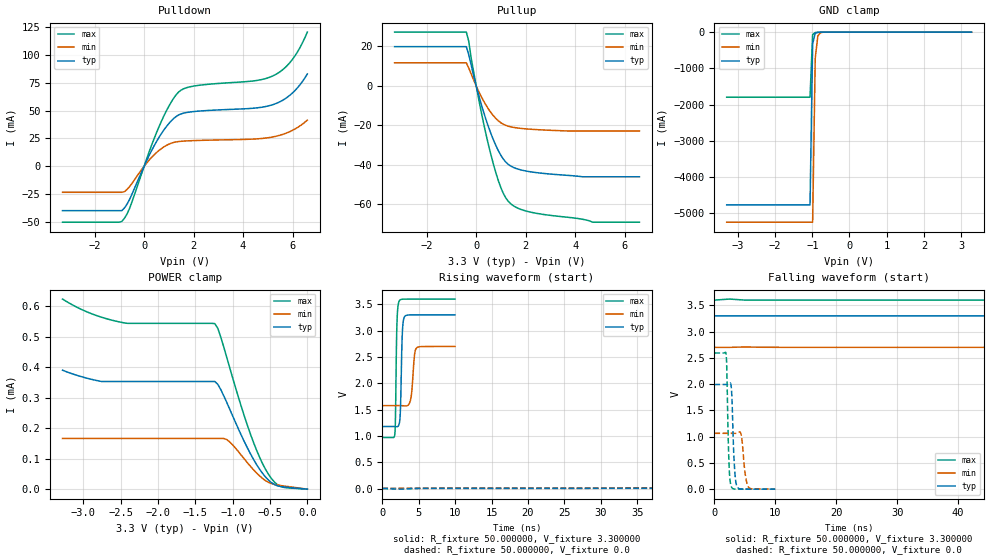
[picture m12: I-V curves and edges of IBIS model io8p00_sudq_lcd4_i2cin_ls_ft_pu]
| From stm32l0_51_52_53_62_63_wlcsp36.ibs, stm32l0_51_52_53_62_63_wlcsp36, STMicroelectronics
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|   Model io8p00_sudq_lcd4_i2cin_ls_ft_pu
[Model]  io8p00_sudq_lcd4_i2cin_ls_ft_pu
Model_type I/O
Polarity   Non-Inverting
Enable   Active-Low
Vinl =   0.990000V
Vinh =   2.310000V
Vmeas =  1.650000V
Cref =   50.000000pF
Rref =   100.000000M
Vref =   0.0V
C_comp   2.499500pF   2.460800pF   2.557800pF
[Temperature Range]   25.000000   0.125000k   -40.000000
[Pullup Reference]   3.300000V   2.700000V   3.600000V
[Pulldown Reference]   0.0V   0.0V   0.0V
[POWER Clamp Reference]   3.300000V   2.700000V   3.600000V
[GND Clamp Reference]   0.0V   0.0V   0.0V
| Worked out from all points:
|   slope of the pulldown table from 0 to 0.495 V, typ, clamps not added: 22.6 ohm
|   slope of the pullup table from 0 to 0.495 V, typ, clamps not added: 23.9 ohm
|   GND clamp passes 1 mA (typ) near -0.64 V on its own axis
|   rising waveform, R_fixture 50.000000, V_fixture 3.300000: 20-80 % time 216ps typ, 364ps min, 175ps max; typ from 1.18 V to 3.3 V
|   rising waveform, R_fixture 50.000000, V_fixture 0.0: 20-80 % time 204ns typ, 424ns min, 99.3ns max; typ from 0.001 V to 1.99 V
|   falling waveform, R_fixture 50.000000, V_fixture 3.300000: 20-80 % time 192ns typ, 381ns min, 105ns max; typ from 3.3 V to 1.18 V
|   falling waveform, R_fixture 50.000000, V_fixture 0.0: 20-80 % time 387ps typ, 554ps min, 311ps max; typ from 1.99 V to 0.001 V
[Pulldown]
|Voltage   I(typ)   I(min)   I(max)
-3.3V     -39.83mA   -23.36mA   -50.2mA
-900mV    -39.83mA   -23.36mA   -49.52mA
-600mV    -30.28mA   -18.59mA   -38.45mA
100mV     4.867mA    2.821mA    6.48mA
600mV     25.85mA    14.17mA    35.39mA
1V        38.33mA    19.81mA    53.88mA
1.4V      46.1mA     22.18mA    66.72mA
2V        49.07mA    23.02mA    71.93mA
4.5V      52.25mA    24.5mA     76.81mA
5.2V      55.25mA    26.31mA    81.02mA
6V        65.79mA    32.24mA    95.96mA
6.6V      82.83mA    41.41mA    120.4mA
[Pullup]
|Voltage   I(typ)   I(min)   I(max)
-3.3V     19.9mA     11.73mA    27.27mA
-400mV    19.9mA     11.73mA    27.27mA
-300mV    15.74mA    8.978mA    22.52mA
-200mV    10.44mA    5.968mA    13.84mA
200mV     -9.115mA   -5.294mA   -12.98mA
600mV     -24.29mA   -13.56mA   -35.12mA
1V        -35.2mA    -18.69mA   -51.63mA
1.2V      -38.62mA   -19.99mA   -56.79mA
1.4V      -40.6mA    -20.72mA   -59.71mA
2.2V      -43.48mA   -21.92mA   -63.91mA
4.7V      -46mA      -22.8mA    -69mA
6.6V      -46mA      -22.8mA    -69mA
[GND_clamp]
|Voltage   I(typ)   I(min)   I(max)
-3.3V     -4.766A    -5.244A    -1.797A
-1.06V    -4.766A    -5.244A    -1.797A
-990mV    -326.4mA   -5.244A    -67.85mA
-920mV    -28.83mA   -721.7mA   -11.08mA
-850mV    -6.686mA   -104.1mA   -6.707mA
-780mV    -3.552mA   -17.28mA   -4.326mA
-500mV    -59.41uA   -172uA     -34.91uA
3.28V     0A         0A         0A
[POWER_clamp]
|Voltage   I(typ)   I(min)   I(max)
-3.28V    390.5uA    166.4uA    624.1uA
-2.76V    353.6uA    166.4uA    564.7uA
-2.44V    353.6uA    166.4uA    545.3uA
-1.24V    353.6uA    166.4uA    543.5uA
-1.2V     344.2uA    166.4uA    528.2uA
-1.16V    327.1uA    166.4uA    499.5uA
-1.04V    262.6uA    155.2uA    398.8uA
-760mV    115.1uA    74.4uA     179.3uA
-560mV    39.87uA    27.94uA    65.07uA
-440mV    15uA       15.53uA    23.15uA
-360mV    8.745uA    12.05uA    9.091uA
0V        0A         0A         0A
[Ramp]
| variable   typ   min   max
dV/dt_r  1.19492/0.20344u   0.61283/0.42621u   1.55547/99.16188n
dV/dt_f  1.27224/0.19134u   0.63582/0.38119u   1.57816/0.10502u
R_load = 50.000000
[Rising Waveform]
R_fixture= 50.000000
V_fixture= 3.300000
V_fixture_min= 2.700000
V_fixture_max= 3.600000
|time   V(typ)   V(min)   V(max)
0s        1.178V     1.575V     969.7mV
1.702ns   1.177V     1.575V     1.018V
2.002ns   1.174V     1.575V     3.123V
2.322ns   1.235V     1.575V     3.563V
2.482ns   1.505V     1.576V     3.587V
2.743ns   2.948V     1.574V     3.597V
3.003ns   3.253V     1.571V     3.598V
3.884ns   3.299V     1.691V     3.599V
4.725ns   3.3V       2.675V     3.6V
9.97ns    3.3V       2.7V       3.6V
[Rising Waveform]
R_fixture= 50.000000
V_fixture= 0.0
V_fixture_min= 0.0
V_fixture_max= 0.0
|time   V(typ)   V(min)   V(max)
0s        1.061mV    1.817mV    656.1uV
50.05ns   4.344mV    4.548mV    94.15mV
100.1ns   82.31mV    4.577mV    928.9mV
165.2ns   466.8mV    10.16mV    1.944V
205.2ns   757.5mV    21.01mV    2.299V
252.8ns   1.082V     58.36mV    2.483V
362.9ns   1.608V     205.7mV    2.576V
503ns     1.883V     450.2mV    2.591V
878.4ns   1.99V      923.1mV    2.593V
1.246us   1.993V     1.064V     2.593V
[Falling Waveform]
R_fixture= 50.000000
V_fixture= 3.300000
V_fixture_min= 2.700000
V_fixture_max= 3.600000
|time   V(typ)   V(min)   V(max)
0s        3.3V       2.7V       3.6V
82.58ns   3.3V       2.7V       3.49V
150.2ns   3.19V      2.7V       2.488V
212.7ns   2.837V     2.697V     1.577V
247.7ns   2.596V     2.687V     1.236V
285.3ns   2.326V     2.665V     1.083V
390.4ns   1.64V      2.552V     998.5mV
490.5ns   1.343V     2.387V     980mV
868.4ns   1.192V     1.749V     970.2mV
1.246us   1.178V     1.575V     969.7mV
[Falling Waveform]
R_fixture= 50.000000
V_fixture= 0.0
V_fixture_min= 0.0
V_fixture_max= 0.0
|time   V(typ)   V(min)   V(max)
0s        1.993V     1.064V     2.593V
1.922ns   1.993V     1.064V     2.563V
2.022ns   1.992V     1.064V     2.306V
2.382ns   1.997V     1.064V     508.3mV
2.783ns   1.914V     1.064V     46.19mV
3.243ns   511.2mV    1.064V     4.312mV
3.664ns   62.27mV    1.066V     1.499mV
4.384ns   3.036mV    1.036V     992.7uV
5.526ns   1.319mV    50.21mV    796.2uV
9.97ns    1.061mV    1.817mV    656.1uV
